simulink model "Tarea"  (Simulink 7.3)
settings: Solver=ode45  StartTime=0.0  StopTime=1.6  MaxStep=Ts  RelTol=1e-4
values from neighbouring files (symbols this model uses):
  Idref = 6    [initial.m]
  Iqref = 8    [initial.m]
  Ki = 421    [initial.m]
  Kp = 23.63    [initial.m]
  L0 = 0.4058    [initial.m]
  Lr = 0.4186    [initial.m]
  Ls = 0.4186    [initial.m]
  Sig = 0.06022    [initial.m]
  Tr = Lr/Rr    (= 0.190272727273)    [initial.m]
  Ts = 1e-6    (= 1e-06)    [initial.m]
  Vmax = 1200    [initial.m]
  wr = 2*pi*30    (= 188.495559215)    [initial.m]    (also in MIJA.m = Viz(4))

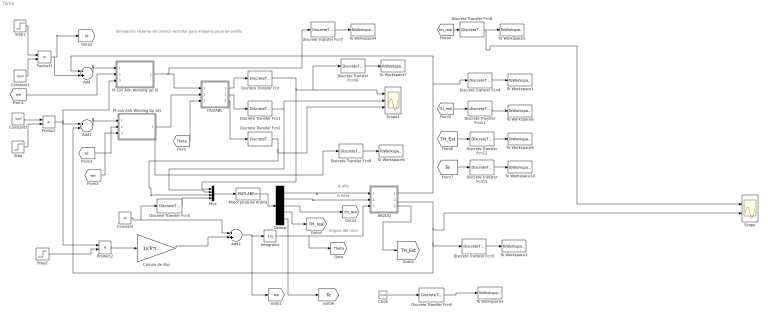
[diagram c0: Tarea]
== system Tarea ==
  note: Simulaciòn sistema de control vectorial para màquina jaula de ardilla
  note: Is alfa
  note: Is Beta
  note: Angulo del rotor
  AB2DQ : Subsystem
  Add : Sum  Inputs=-+  OutDataType=sfix(16)  OutScaling=2^-10
  Add1 : Sum  Inputs=+-  OutDataType=sfix(16)  OutScaling=2^-10
  Add2 : Sum  OutDataType=sfix(16)  OutScaling=2^-10
  Calculo de Slip : Gain  Gain=1/(Tr*Idref)  ParameterDataType=sfix(16)  ParameterScaling=2^0  OutDataType=sfix(16)  OutScaling=2^0
  Clock : Clock
  Constant : Constant  Value=wr  OutDataType=sfix(16)  OutScaling=2^0
  Constant1 : Constant  Value=Idref  OutDataType=sfix(16)  OutScaling=2^0
  Constant2 : Constant  Value=Iqref  OutDataType=sfix(16)  OutScaling=2^0
  DQ2ABC : Subsystem
  Demux : Demux  Outputs=5
  Discrete Transfer Fcn{,1..13} (14 alike) : DiscreteTransferFcn  Denominator=[1]  SampleTime=Ts
  Integrator : Integrator
  Motor Jaula de Ardilla : MATLABFcn  MATLABFcn=MIJA  OutputDimensions=5
  Mux : Mux
  PI con Anti Winding Up Id : Subsystem
  PI con Anti Winding Up Id1 : Subsystem
  Product : Product  OutDataType=fixdt(1, 16)  OutScaling=2^0
  Product1 : Product  OutDataType=fixdt(1, 16)  OutScaling=2^0
  Product2 : Product  OutDataType=fixdt(1, 16)  OutScaling=2^0
  Scope : Scope  NumInputPorts=2
  Scope1 : Scope  NumInputPorts=3
  Step : Step  Time=0.7  Before=1  After=2  SampleTime=0
  Step1 : Step  Time=5  Before=1  After=2  SampleTime=0
  Step2 : Step  Time=0  Before=1  After=0.5  SampleTime=0
  To Workspace1 : ToWorkspace  VariableName=Id  SampleTime=-1  SaveFormat=Array
  To Workspace10 : ToWorkspace  VariableName=Te  SampleTime=-1  SaveFormat=Array
  To Workspace2 : ToWorkspace  VariableName=Iq  SampleTime=-1  SaveFormat=Array
  To Workspace3 : ToWorkspace  VariableName=time  SampleTime=-1  SaveFormat=Array
  To Workspace4 : ToWorkspace  VariableName=Vd  SampleTime=-1  SaveFormat=Array
  To Workspace5 : ToWorkspace  VariableName=Im_real  SampleTime=-1  SaveFormat=Array
  To Workspace6 : ToWorkspace  VariableName=Vq  SampleTime=-1  SaveFormat=Array
  To Workspace7 : ToWorkspace  VariableName=Va  SampleTime=-1  SaveFormat=Array
  To Workspace8 : ToWorkspace  VariableName=TH_real  SampleTime=-1  SaveFormat=Array
  To Workspace9 : ToWorkspace  VariableName=TH_Est  SampleTime=-1  SaveFormat=Array
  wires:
  Constant/1 -> Add2/1, Discrete Transfer Fcn3/1
  Add/1 -> PI con Anti Winding Up Id/1(Error)
  Add1/1 -> PI con Anti Winding Up Id1/1(Error)
  Add2/1 -> Integrator/1, [we]
  Calculo de Slip/1 -> Add2/2
  Demux/1 -> AB2DQ/1(Ialfa)
  Demux/2 -> AB2DQ/2(Ibeta)
  Integrator/1 -> AB2DQ/3(Theta), [Theta]
  AB2DQ/1(Id) -> Add/1, Discrete Transfer Fcn4/1
  AB2DQ/2(Iq) -> Scope/2, Add1/2, Discrete Transfer Fcn5/1
  [Theta] -> DQ2ABC/3(Theta)
  DQ2ABC/1(Va) -> Discrete Transfer Fcn/1
  DQ2ABC/2(Vb) -> Discrete Transfer Fcn1/1
  DQ2ABC/3(Vc) -> Discrete Transfer Fcn2/1
  Discrete Transfer Fcn3/1 -> Mux/4
  Discrete Transfer Fcn2/1 -> Scope1/3, Mux/3
  Discrete Transfer Fcn1/1 -> Scope1/2, Mux/2
  Discrete Transfer Fcn/1 -> Mux/1, Scope1/1, Discrete Transfer Fcn10/1
  PI con Anti Winding Up Id/1(Vd) -> DQ2ABC/1(Vd), Discrete Transfer Fcn7/1
  PI con Anti Winding Up Id1/1(Vq) -> DQ2ABC/2(Vq), Discrete Transfer Fcn9/1
  Discrete Transfer Fcn4/1 -> To Workspace1/1
  Discrete Transfer Fcn5/1 -> To Workspace2/1
  Discrete Transfer Fcn6/1 -> To Workspace3/1
  Clock/1 -> Discrete Transfer Fcn6/1
  Discrete Transfer Fcn7/1 -> To Workspace4/1
  Discrete Transfer Fcn9/1 -> To Workspace6/1
  Motor Jaula de Ardilla/1 -> Demux/1
  Mux/1 -> Motor Jaula de Ardilla/1
  Discrete Transfer Fcn10/1 -> To Workspace7/1
  Constant2/1 -> Product/1
  Product/1 -> Add1/1, PI con Anti Winding Up Id/3(Iq), Product2/1
  Step/1 -> Product/2
  [we] -> PI con Anti Winding Up Id/2(We)
  [we] -> PI con Anti Winding Up Id1/3(We)
  [Id] -> PI con Anti Winding Up Id1/2(Id)
  Demux/3 -> [Im_real]
  [Im_real] -> Discrete Transfer Fcn8/1
  Discrete Transfer Fcn8/1 -> To Workspace5/1, Scope/1
  Demux/4 -> [TH_real]
  [TH_real] -> Discrete Transfer Fcn11/1
  Discrete Transfer Fcn11/1 -> To Workspace8/1
  AB2DQ/3(Theta_e) -> [TH_Est]
  [TH_Est] -> Discrete Transfer Fcn12/1
  Discrete Transfer Fcn12/1 -> To Workspace9/1
  Demux/5 -> [Te]
  [Te] -> Discrete Transfer Fcn13/1
  Discrete Transfer Fcn13/1 -> To Workspace10/1
  Constant1/1 -> Product1/2
  Product1/1 -> [Id], Add/2
  Step1/1 -> Product1/1
  Product2/1 -> Calculo de Slip/1
  Step2/1 -> Product2/2

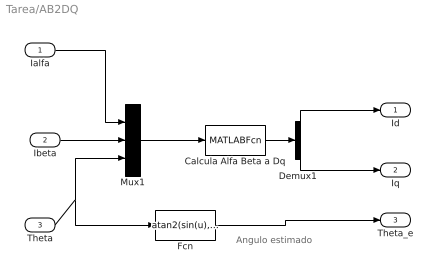
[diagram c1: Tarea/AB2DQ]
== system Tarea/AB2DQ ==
  note: Angulo estimado
  Ialfa : Inport  OutDataType=sfix(16)  OutScaling=2^0
  Ibeta : Inport  Port=2  OutDataType=sfix(16)  OutScaling=2^0
  Theta : Inport  Port=3  OutDataType=sfix(16)  OutScaling=2^0
  Calcula Alfa Beta a Dq : MATLABFcn  MATLABFcn=AB2DQ  OutputDimensions=2
  Demux1 : Demux  Outputs=2
  Fcn : Fcn  Expr=atan2(sin(u),cos(u))
  Mux1 : Mux  Inputs=3
  Id : Outport  OutDataType=sfix(16)  OutScaling=2^0
  Iq : Outport  Port=2  OutDataType=sfix(16)  OutScaling=2^0
  Theta_e : Outport  Port=3  OutDataType=sfix(16)  OutScaling=2^0
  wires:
  Mux1/1 -> Calcula Alfa Beta a Dq/1
  Calcula Alfa Beta a Dq/1 -> Demux1/1
  Ialfa/1 -> Mux1/1
  Demux1/1 -> Id/1
  Ibeta/1 -> Mux1/2
  Demux1/2 -> Iq/1
  Theta/1 -> Mux1/3, Fcn/1
  Fcn/1 -> Theta_e/1

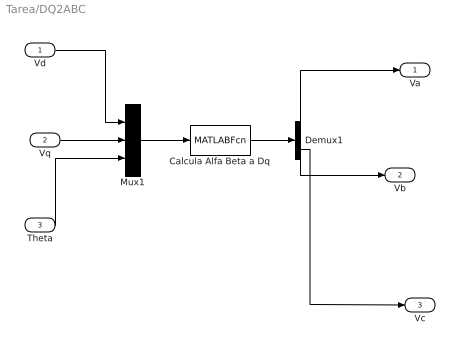
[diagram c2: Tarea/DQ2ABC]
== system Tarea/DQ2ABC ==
  Vd : Inport  OutDataType=sfix(16)  OutScaling=2^0
  Vq : Inport  Port=2  OutDataType=sfix(16)  OutScaling=2^0
  Theta : Inport  Port=3  OutDataType=sfix(16)  OutScaling=2^0
  Calcula Alfa Beta a Dq : MATLABFcn  MATLABFcn=DQ2ABC  OutputDimensions=3
  Demux1 : Demux  Outputs=3
  Mux1 : Mux  Inputs=3
  Va : Outport  OutDataType=sfix(16)  OutScaling=2^0
  Vb : Outport  Port=2  OutDataType=sfix(16)  OutScaling=2^0
  Vc : Outport  Port=3  OutDataType=sfix(16)  OutScaling=2^0
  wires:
  Theta/1 -> Mux1/3
  Demux1/2 -> Vb/1
  Vq/1 -> Mux1/2
  Demux1/1 -> Va/1
  Vd/1 -> Mux1/1
  Calcula Alfa Beta a Dq/1 -> Demux1/1
  Mux1/1 -> Calcula Alfa Beta a Dq/1
  Demux1/3 -> Vc/1

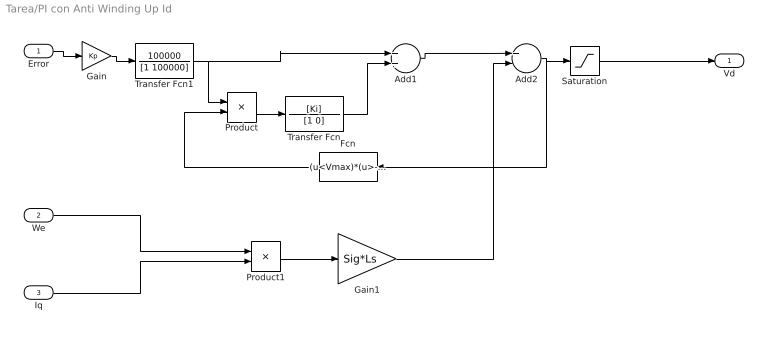
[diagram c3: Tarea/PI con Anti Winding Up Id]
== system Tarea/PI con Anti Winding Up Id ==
  Error : Inport  OutDataType=sfix(16)  OutScaling=2^0
  We : Inport  Port=2  OutDataType=sfix(16)  OutScaling=2^0
  Iq : Inport  Port=3  OutDataType=sfix(16)  OutScaling=2^0
  Add1 : Sum  OutDataType=sfix(16)  OutScaling=2^-10
  Add2 : Sum  Inputs=+-  OutDataType=sfix(16)  OutScaling=2^-10
  Fcn : Fcn  Expr=(u<Vmax)*(u>-Vmax)
  Gain : Gain  Gain=Kp  ParameterDataType=sfix(16)  ParameterScaling=2^0  OutDataType=sfix(16)  OutScaling=2^0
  Gain1 : Gain  Gain=Sig*Ls  ParameterDataType=sfix(16)  ParameterScaling=2^0  OutDataType=sfix(16)  OutScaling=2^0
  Product : Product  OutDataType=sfix(16)  OutScaling=2^0
  Product1 : Product  OutDataType=sfix(16)  OutScaling=2^0
  Saturation : Saturate  UpperLimit=Vmax  LowerLimit=-Vmax
  Transfer Fcn : TransferFcn  Numerator=[Ki]  Denominator=[1 0]
  Transfer Fcn1 : TransferFcn  Numerator=100000  Denominator=[1 100000]
  Vd : Outport  OutDataType=sfix(16)  OutScaling=2^0
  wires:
  Transfer Fcn/1 -> Add1/2
  Product/1 -> Transfer Fcn/1
  Add1/1 -> Add2/1
  Fcn/1 -> Product/2
  Error/1 -> Gain/1
  Saturation/1 -> Vd/1
  Gain/1 -> Transfer Fcn1/1
  Transfer Fcn1/1 -> Add1/1, Product/1
  Add2/1 -> Saturation/1, Fcn/1
  We/1 -> Product1/1
  Iq/1 -> Product1/2
  Product1/1 -> Gain1/1
  Gain1/1 -> Add2/2

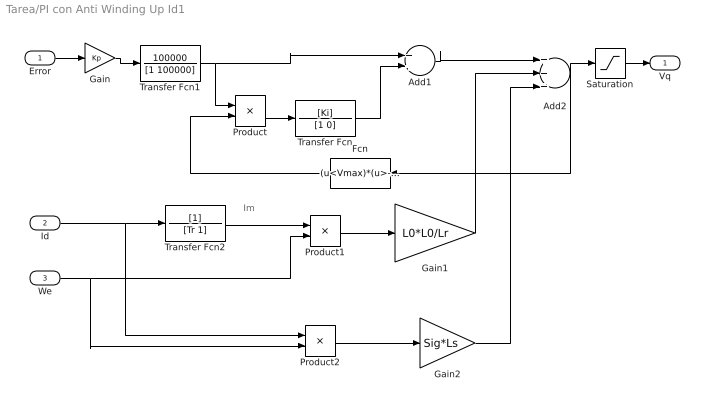
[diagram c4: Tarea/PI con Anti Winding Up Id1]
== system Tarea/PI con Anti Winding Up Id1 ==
  note: Im
  Error : Inport  OutDataType=sfix(16)  OutScaling=2^0
  Id : Inport  Port=2  OutDataType=sfix(16)  OutScaling=2^0
  We : Inport  Port=3  OutDataType=sfix(16)  OutScaling=2^0
  Add1 : Sum  OutDataType=sfix(16)  OutScaling=2^-10
  Add2 : Sum  Inputs=+++  OutDataType=sfix(16)  OutScaling=2^-10
  Fcn : Fcn  Expr=(u<Vmax)*(u>-Vmax)
  Gain : Gain  Gain=Kp  ParameterDataType=sfix(16)  ParameterScaling=2^0  OutDataType=sfix(16)  OutScaling=2^0
  Gain1 : Gain  Gain=L0*L0/Lr  ParameterDataType=sfix(16)  ParameterScaling=2^0  OutDataType=sfix(16)  OutScaling=2^0
  Gain2 : Gain  Gain=Sig*Ls  ParameterDataType=sfix(16)  ParameterScaling=2^0  OutDataType=sfix(16)  OutScaling=2^0
  Product : Product  OutDataType=sfix(16)  OutScaling=2^0
  Product1 : Product  OutDataType=sfix(16)  OutScaling=2^0
  Product2 : Product  OutDataType=sfix(16)  OutScaling=2^0
  Saturation : Saturate  UpperLimit=Vmax  LowerLimit=-Vmax
  Transfer Fcn : TransferFcn  Numerator=[Ki]  Denominator=[1 0]
  Transfer Fcn1 : TransferFcn  Numerator=100000  Denominator=[1 100000]
  Transfer Fcn2 : TransferFcn  Denominator=[Tr 1]
  Vq : Outport  OutDataType=sfix(16)  OutScaling=2^0
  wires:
  Transfer Fcn1/1 -> Product/1, Add1/1
  Gain/1 -> Transfer Fcn1/1
  Saturation/1 -> Vq/1
  Error/1 -> Gain/1
  Fcn/1 -> Product/2
  Add1/1 -> Add2/1
  Product/1 -> Transfer Fcn/1
  Transfer Fcn/1 -> Add1/2
  Id/1 -> Transfer Fcn2/1, Product2/1
  Add2/1 -> Saturation/1, Fcn/1
  Transfer Fcn2/1 -> Product1/1
  We/1 -> Product1/2, Product2/2
  Product1/1 -> Gain1/1
  Product2/1 -> Gain2/1
  Gain1/1 -> Add2/2
  Gain2/1 -> Add2/3
